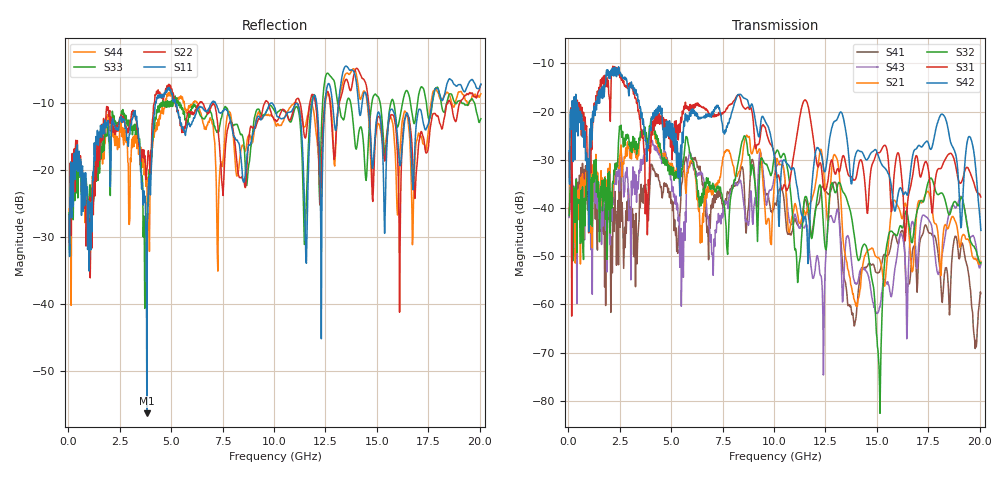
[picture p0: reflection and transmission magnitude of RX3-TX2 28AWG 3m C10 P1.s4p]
! FILE: O:\PROJECTS\SI-2007-05-003 3m Eyemax Qual\XT\FD\RX3-TX2 28AWG 3m C10 P1.s4p
# MHZ S RI R 50.00
! FREQ  S11  S12  S13  S14
!  S21  S22  S23  S24
!  S31  S32  S33  S34
!  S41  S42  S43  S44
!  REAL  IMAG  REAL  IMAG  REAL  IMAG  REAL  IMAG
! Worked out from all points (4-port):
!   801 points, 50 MHz to 20.05 GHz, reference 50 ohm
!   strongest paths, dB at 50 MHz, 5.05 GHz, 10.05 GHz, 15.05 GHz, 20.05 GHz:
!     S42: -28.1, -25.9, -29.9, -29.0, -44.6
!     S31: -28.5, -30.0, -29.7, -28.5, -37.7
!     S32: -41.6, -31.6, -28.6, -69.3, -51.3
!     S21: -40.9, -30.8, -34.0, -50.3, -51.1
!     S43: -41.9, -36.6, -32.7, -61.7, -51.6
!     S41: -41.5, -38.7, -38.9, -53.5, -57.7
!   lowest |S11| = -56.4 dB at 3.825 GHz (marker M1), VSWR 1.00, Z = 49.9 + j0.072 ohm
!   |S11| at or under -10 dB: start of sweep to 4.245 GHz; 7.157 GHz to 11.86 GHz (4.706 GHz wide, 49.5 % of centre); 14.55 GHz to 17.68 GHz (3.128 GHz wide, 19.4 % of centre)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
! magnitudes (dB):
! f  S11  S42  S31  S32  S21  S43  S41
! 50 MHz  -26.8  -28.1  -28.5  -41.6  -40.9  -41.9  -41.5
! 3.825 GHz  -56.4  -30.3  -41.4  -26.0  -26.9  -28.6  -37.1
! 11.62 GHz  -26.1  -47.6  -18.3  -38.5  -40.0  -44.3  -40.1
! 13.2 GHz  -8.3  -20.3  -32.2  -34.8  -34.5  -44.7  -43.6
! 15.1 GHz  -11.5  -29.6  -28.6  -72.7  -50.4  -61.2  -53.3
! 17.57 GHz  -12.0  -27.7  -34.9  -33.9  -37.5  -42.9  -45.2
! 20.05 GHz  -7.2  -44.6  -37.7  -51.3  -51.1  -51.6  -57.7
